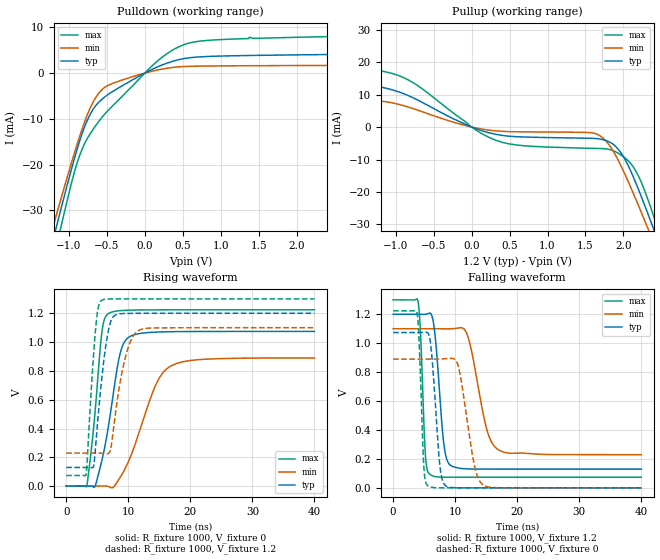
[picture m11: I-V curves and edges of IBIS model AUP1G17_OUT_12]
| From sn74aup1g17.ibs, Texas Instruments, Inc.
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[Model]   AUP1G17_OUT_12
Model_type  Output
Vref =   0
Rref =   1E6
Cref =   30p
Vmeas =   0.6
| variable   typ   min   max
C_comp   2.85pF   2.12pF   3.93pF
| C_pullup   3.03pF   2.12pF   3.93pF
| C_pulldown   2.67pF   2.23pF   3.17pF
[Temperature Range]   40   100   -40
| Ambient temperature   25   85   -40
[Voltage range]   1.2   1.1   1.3
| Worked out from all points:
|   slope of the pulldown table from 0 to 0.18 V, typ, clamps not added: 125 ohm
|   slope of the pullup table from 0 to 0.18 V, typ, clamps not added: 123 ohm
|   rising waveform, R_fixture 1000, V_fixture 0: 20-80 % time 2.44ns typ, 4.44ns min, 1.5ns max; typ from 0 V to 1.07 V
|   falling waveform, R_fixture 1000, V_fixture 1.2: 20-80 % time 1.16ns typ, 2.36ns min, 657ps max; typ from 1.2 V to 0.129 V
|   rising waveform, R_fixture 1000, V_fixture 1.2: 20-80 % time 1.55ns typ, 2.1ns min, 1.1ns max; typ from 0.129 V to 1.2 V
|   falling waveform, R_fixture 1000, V_fixture 0: 20-80 % time 1.05ns typ, 1.91ns min, 612ps max; typ from 1.07 V to 0 V
[Pulldown]
| AUP1G17_OUT_12
|   Voltage   I(typ)   I(min)   I(max)
-3.6V     -203.6mA   -186.6mA   -224.6mA
-1.215V   -36.77mA   -33.88mA   -41.55mA
-1.165V   -33.49mA   -30.92mA   -37.89mA
-1.12V    -30.57mA   -28.28mA   -34.63mA
-1.08V    -28mA      -25.95mA   -31.76mA
-930mV    -18.76mA   -17.53mA   -21.68mA
-820mV    -12.87mA   -11.86mA   -16.33mA
-695mV    -8.261mA   -6.747mA   -12.62mA
-580mV    -5.938mA   -3.862mA   -9.962mA
160mV     1.298mA    643.5uA    2.533mA
610mV     3.376mA    1.481mA    6.659mA
7.2V      4.761mA    1.852mA    9.574mA
[Pullup]
| AUP1G17_OUT_12
|   Voltage   I(typ)   I(min)   I(max)
-3.6V     26.64mA    8.226mA    37.8mA
-3.065V   21.41mA    10.49mA    30.92mA
-2.05V    13.06mA    7.529mA    19.66mA
-955mV    10.79mA    6.951mA    15.81mA
400mV     -2.561mA   -1.314mA   -4.679mA
1.61V     -3.491mA   -1.891mA   -6.566mA
1.87V     -5.387mA   -7.563mA   -7.321mA
2.095V    -13.49mA   -18.49mA   -11.17mA
2.33V     -27.16mA   -31.66mA   -22.8mA
2.44V     -34.07mA   -38.08mA   -30.25mA
2.51V     -38.55mA   -42.22mA   -35.17mA
7.2V      -371mA     -348.5mA   -398.6mA
[Ramp]
| AUP1G17_OUT_12
| variable   typ   min   max
dV/dt_r   0.65/2.47E-09   0.54/4.51E-09   0.74/1.51E-09
dV/dt_f   0.65/1.17E-09   0.53/2.38E-09   0.74/6.65E-10
R_load = 1000
[Rising Waveform]
| AUP1G17_OUT_12
R_fixture =   1000
C_fixture =   0
L_fixture =   0
V_fixture =   0
V_fixture_min = 0
V_fixture_max = 0
|   Time   V(typ)   V(min)   V(max)
0s        17.04nV    106.6nV    899pV
3.305ns   178.9uV    -14.19uV   2.306mV
4.59ns    -5.254mV   59.02uV    487mV
5.725ns   175.5mV    592.6uV    1.061V
6.78ns    410.4mV    -2.16mV    1.197V
8.395ns   863.3mV    41.14mV    1.217V
9.43ns    1.004V     117.3mV    1.22V
14.35ns   1.069V     694.6mV    1.224V
16.7ns    1.072V     829.6mV    1.224V
40ns      1.074V     889.8mV    1.224V
[Falling Waveform]
| AUP1G17_OUT_12
R_fixture =   1000
C_fixture =   0
L_fixture =   0
V_fixture =   1.2
V_fixture_min = 1.1
V_fixture_max = 1.3
|   Time   V(typ)   V(min)   V(max)
0s        1.2V       1.1V       1.3V
4.005ns   1.2V       1.1V       1.291V
5.2ns     1.2V       1.1V       231.7mV
5.93ns    1.208V     1.1V       93.16mV
6.75ns    1.058V     1.1V       77.85mV
8.215ns   291mV      1.099V     73.81mV
9.24ns    155.6mV    1.099V     73.59mV
11.9ns    131mV      1.063V     73.54mV
16.93ns   129.5mV    264.2mV    73.54mV
40ns      129.5mV    229.3mV    73.54mV
[Rising Waveform]
| AUP1G17_OUT_12
R_fixture =   1000
C_fixture =   0
L_fixture =   0
V_fixture =   1.2
V_fixture_min = 1.1
V_fixture_max = 1.3
|   Time   V(typ)   V(min)   V(max)
0s        129.5mV    229.3mV    73.54mV
3.185ns   129.6mV    229.4mV    78.19mV
4.455ns   148.8mV    229.5mV    941.7mV
5.04ns    435.4mV    229.3mV    1.21V
5.695ns   734.6mV    228.1mV    1.29V
6.595ns   1.035V     224.9mV    1.298V
7.385ns   1.163V     320.1mV    1.299V
9.385ns   1.198V     869.5mV    1.3V
11.65ns   1.2V       1.08V      1.3V
40ns      1.2V       1.1V       1.3V
[Falling Waveform]
| AUP1G17_OUT_12
R_fixture =   1000
C_fixture =   0
L_fixture =   0
V_fixture =   0
V_fixture_min = 0
V_fixture_max = 0
|   Time   V(typ)   V(min)   V(max)
0s        1.074V     889.8mV    1.224V
3.855ns   1.074V     889.8mV    1.211V
4.95ns    1.075V     889.7mV    148.5mV
5.585ns   1.071V     889.7mV    14.9mV
7.56ns    145mV      890.7mV    160.7uV
8.495ns   13.25mV    893.1mV    20.25uV
10.48ns   360.4uV    844.9mV    735.9nV
13.08ns   11.63uV    158.7mV    178.3nV
14.56ns   2.518uV    19.05mV    -31.3nV
40ns      -98.75nV   328.7nV    -49.62nV
